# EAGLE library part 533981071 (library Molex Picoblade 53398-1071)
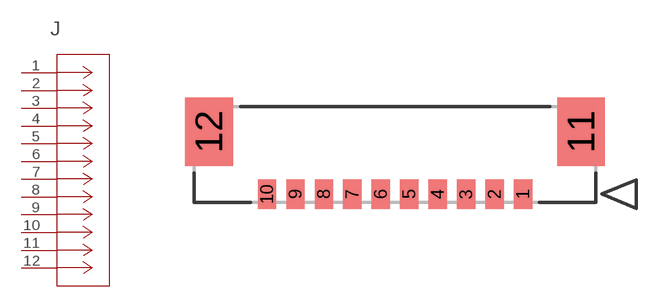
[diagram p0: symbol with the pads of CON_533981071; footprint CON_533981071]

Designator prefix J

## 533981071 (COPYRIGHT: Copyright (C) 2022 Ultra Librarian. All rights reserved.; MANUFACTURER_PART_NUMBER: 533981071; MFR_NAME: Molex Connector Corporation)  [CON_533981071]
1  1  pas
2  2  pas
3  3  pas
4  4  pas
5  5  pas
6  6  pas
7  7  pas
8  8  pas
9  9  pas
10  10  pas
11  11  pas
12  12  pas

## Footprint CON_533981071 (pad centres in mm)
smd 0.8 x 1.3: 1 0,0; 2 -1.25,0; 3 -2.5,0; 4 -3.75,0; 5 -5,0; 6 -6.25,0; 7 -7.5,0; 8 -8.75,0; 9 -10,0; 10 -11.25,0
smd 2.1 x 3: 11 2.55,2.75; 12 -13.8,2.75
